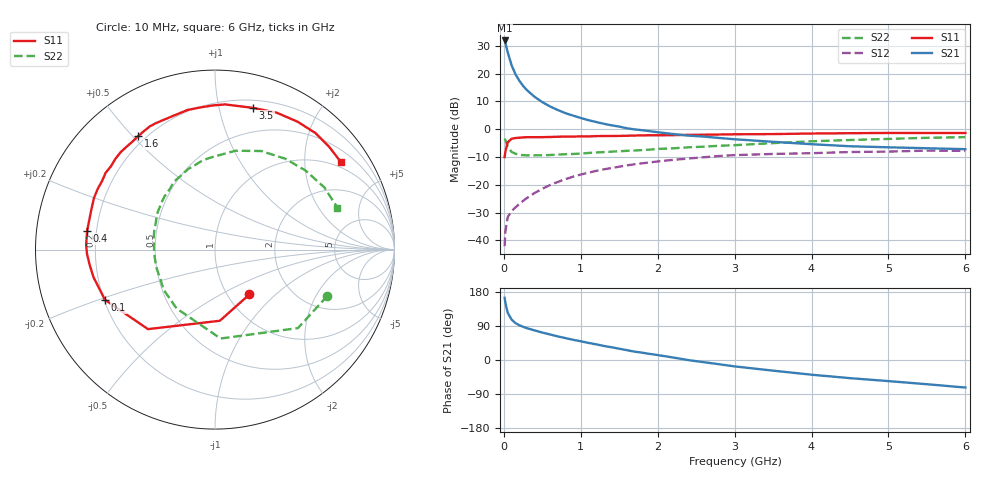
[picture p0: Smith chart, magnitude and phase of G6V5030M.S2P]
! SIEMENS Small Signal Semiconductors
! BFG193
! Si NPN RF Bipolar Junction Transistor in SOT223
! VCE = 0.5 V  IC = 30 mA
! Common Emitter S-Parameters:  August  1996
# GHz  S  MA  R  50
!  f  S11  S21  S12  S22
! GHz  MAG  ANG  MAG  ANG  MAG  ANG  MAG  ANG
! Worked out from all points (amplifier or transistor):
!   36 points, 10 MHz to 6 GHz, reference 50 ohm
!   highest |S21| = 31.9 dB at 10 MHz (marker M1)
!   |S21| within 3 dB of that: start of sweep to 38.99 MHz
!   unconditionally stable (mu >= 1): 275.1 MHz to end of sweep
!   at 250 MHz: K = 0.97, MSG = 20.7 dB, |S12| = -25.8 dB
!   at 1.4 GHz: K = 1.17, MAG = 5.2 dB, |S12| = -14.0 dB
!   at 6 GHz: K = 1.06, MAG = -1.1 dB, |S12| = -7.8 dB
!   S11 on the Smith chart (normalised r, x): 10 MHz: 1.26, -0.70; 100 MHz: 0.20, -0.21; 400 MHz: 0.16, +0.07; 1.6 GHz: 0.17, +0.52; 3.5 GHz: 0.27, +1.27; 6 GHz: 0.83, +2.99
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0.01  0.315 -52.4  39.42 164.1  0.0079 76.2  0.6771 -22.4
0.02  0.3974 -86.1  35.69 151.1  0.0145 66.8  0.6364 -43.4
0.05  0.5793 -130.1  24.2 124.7  0.0262 48.7  0.4964 -86.4
0.1  0.6736 -155.4  14.22 106.8  0.0337 44.9  0.3915 -123.1
0.15  0.6941 -167.1  9.803 97.5  0.0392 46.2  0.3631 -142.2
0.2  0.7036 -173.1  7.5 91.9  0.0452 49.8  0.3443 -152.8
0.25  0.7137 -178.2  6.017 87.6  0.0515 51.6  0.3415 -161.5
0.3  0.7184 177.9  5.04 84.0  0.0579 53.8  0.3393 -166.9
0.4  0.7201 171.7  3.822 78.1  0.0713 55.8  0.3395 -176.1
0.5  0.7202 166.0  3.069 72.4  0.0849 55.8  0.3402 177.1
0.6  0.7248 161.6  2.57 67.4  0.0992 55.3  0.344 171.8
0.7  0.7329 156.9  2.217 62.3  0.1126 54.3  0.3496 167.0
0.9  0.7361 148.8  1.756 53.4  0.1403 50.7  0.3589 157.8
1.1  0.7426 141.3  1.452 45.1  0.1656 47.0  0.3739 150.6
1.3  0.7556 134.1  1.252 37.1  0.1901 42.4  0.388 142.8
1.6  0.7632 124.2  1.04 25.9  0.224 34.7  0.409 133.2
2.2  0.7817 106.6  0.82 6.6  0.2815 19.7  0.4535 114.8
2.8  0.8035 90.7  0.696 -11.2  0.33 4.8  0.5036 97.4
3.5  0.8178 74.9  0.594 -28.1  0.3593 -13.1  0.5626 78.3
4.5  0.8482 57.1  0.494 -47.9  0.3891 -31.8  0.64 52.3
5.5  0.8558 42.0  0.455 -63.9  0.4127 -53.0  0.7007 29.7
6  0.8545 34.7  0.438 -72.7  0.4085 -65.2  0.7211 18.9
